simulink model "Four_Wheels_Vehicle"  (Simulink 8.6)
settings: Solver=ode45  StartTime=0.0  StopTime=20  RelTol=1e-3
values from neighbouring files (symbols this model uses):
  beta = 1    [Vehicle_Parameters.m]
  g = 9.81    [Vehicle_Parameters.m]
  H_CoG = 0.700    (= 0.7)    [Vehicle_Parameters.m]
  Hearo = 0.750    (= 0.75)    [Vehicle_Parameters.m]
  Iz = 2480    [Vehicle_Parameters.m]
  Jw = 2.166    [Vehicle_Parameters.m]
  L = 10    [Vehicle_Parameters.m]
  Lf = 1.180    (= 1.18)    [Vehicle_Parameters.m]
  Lr = 1.770    (= 1.77)    [Vehicle_Parameters.m]
  Lw = 1.880    (= 1.88)    [Vehicle_Parameters.m]
  m = 1500    [Vehicle_Parameters.m]
  miu = 0.85    [Vehicle_Parameters.m]
  reff = 0.380    (= 0.38)    [Vehicle_Parameters.m]
undefined symbols (not defined in the file or in its folder): DiscIntNeverNeededParam, Init, Ki, Kp, LowerLimit, sigbuilder_block, Ts, UpperLimit
libraries: simulink x15, powerlib_extras x3
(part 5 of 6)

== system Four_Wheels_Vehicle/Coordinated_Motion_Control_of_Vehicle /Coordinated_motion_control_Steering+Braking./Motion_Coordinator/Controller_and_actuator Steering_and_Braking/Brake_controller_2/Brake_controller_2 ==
  Reference : Inport
  Feedback : Inport  Port=2
  Controller : Subsystem  AncestorBlock=|  DialogController=POWERSYS.PowerSysDialog
      | powerlib_extras/Discrete 
      | Control Blocks/Discrete
      | PI Controller
  Controller1 : Subsystem  AncestorBlock=|  DialogController=POWERSYS.PowerSysDialog
      | powerlib_extras/Discrete 
      | Control Blocks/Discrete
      | PI Controller
  Scope : Scope
  Scope1 : Scope
  Scope2 : Scope  NumInputPorts=2
  Sum1 : Sum  Inputs=-+
  Sum2 : Sum
  Sideslip_Ang : Outport
  Sideslip_Ang1 : Outport  Port=2
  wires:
  Sum2/1 -> Sideslip_Ang1/1, Scope2/2
  Reference/1 -> Sum1/2, Controller1/1(Error)
  Controller1/1(Out) -> Sum2/2
  Feedback/1 -> Sum1/1
  Sum1/1 -> Scope/1, Controller/1(Error)
  Controller/1(Out) -> Sideslip_Ang/1, Scope2/1, Sum2/1, Scope1/1

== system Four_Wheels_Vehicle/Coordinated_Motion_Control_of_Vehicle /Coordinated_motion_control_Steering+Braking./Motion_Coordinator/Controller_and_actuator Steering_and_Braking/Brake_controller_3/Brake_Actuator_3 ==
  input : Inport
  Actuator : Subsystem
  Cut_off_frequency : Constant  Value=10  SampleTime=-1
  output : Outport
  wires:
  input/1 -> Actuator/1(In1)
  Actuator/1(out) -> output/1
  Cut_off_frequency/1 -> Actuator/2(fre)

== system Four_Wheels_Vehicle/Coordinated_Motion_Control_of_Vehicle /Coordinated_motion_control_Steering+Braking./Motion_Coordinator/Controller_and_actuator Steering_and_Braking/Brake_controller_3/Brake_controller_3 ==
  Reference : Inport
  Feedback : Inport  Port=2
  Controller : Subsystem  AncestorBlock=|  DialogController=POWERSYS.PowerSysDialog
      | powerlib_extras/Discrete 
      | Control Blocks/Discrete
      | PI Controller
  Controller1 : Subsystem  AncestorBlock=|  DialogController=POWERSYS.PowerSysDialog
      | powerlib_extras/Discrete 
      | Control Blocks/Discrete
      | PI Controller
  Scope : Scope
  Scope1 : Scope
  Scope2 : Scope  NumInputPorts=2
  Sum1 : Sum  Inputs=-+
  Sum2 : Sum
  Sideslip_Ang : Outport
  Sideslip_Ang1 : Outport  Port=2
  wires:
  Controller/1(Out) -> Scope1/1, Sum2/1, Scope2/1, Sideslip_Ang/1
  Sum1/1 -> Controller/1(Error), Scope/1
  Feedback/1 -> Sum1/1
  Controller1/1(Out) -> Sum2/2
  Reference/1 -> Controller1/1(Error), Sum1/2
  Sum2/1 -> Scope2/2, Sideslip_Ang1/1

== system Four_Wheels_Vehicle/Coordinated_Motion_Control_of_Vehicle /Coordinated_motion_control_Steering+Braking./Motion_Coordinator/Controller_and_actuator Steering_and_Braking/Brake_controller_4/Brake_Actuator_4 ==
  input : Inport
  Actuator : Subsystem
  Cut_off_frequency : Constant  Value=10  SampleTime=-1
  output : Outport
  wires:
  Cut_off_frequency/1 -> Actuator/2(fre)
  Actuator/1(out) -> output/1
  input/1 -> Actuator/1(In1)

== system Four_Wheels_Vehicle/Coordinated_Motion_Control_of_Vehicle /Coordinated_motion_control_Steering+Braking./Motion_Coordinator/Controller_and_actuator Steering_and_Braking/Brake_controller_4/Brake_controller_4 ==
  Reference : Inport
  Feedback : Inport  Port=2
  Controller : Subsystem  AncestorBlock=|  DialogController=POWERSYS.PowerSysDialog
      | powerlib_extras/Discrete 
      | Control Blocks/Discrete
      | PI Controller
  Controller1 : Subsystem  AncestorBlock=|  DialogController=POWERSYS.PowerSysDialog
      | powerlib_extras/Discrete 
      | Control Blocks/Discrete
      | PI Controller
  Scope : Scope
  Scope1 : Scope
  Scope2 : Scope  NumInputPorts=2
  Sum1 : Sum  Inputs=-+
  Sum2 : Sum
  Sideslip_Ang : Outport
  Sideslip_Ang1 : Outport  Port=2
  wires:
  Sum2/1 -> Sideslip_Ang1/1, Scope2/2
  Reference/1 -> Sum1/2, Controller1/1(Error)
  Controller1/1(Out) -> Sum2/2
  Feedback/1 -> Sum1/1
  Sum1/1 -> Scope/1, Controller/1(Error)
  Controller/1(Out) -> Sideslip_Ang/1, Scope2/1, Sum2/1, Scope1/1

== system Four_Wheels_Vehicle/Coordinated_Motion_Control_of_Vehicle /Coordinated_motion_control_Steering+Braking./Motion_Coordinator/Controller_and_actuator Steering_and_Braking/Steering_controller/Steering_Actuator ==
  input : Inport
  Actuator : Subsystem
  Cut_off_frequency : Constant  Value=5  SampleTime=-1
  output : Outport
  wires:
  Cut_off_frequency/1 -> Actuator/2(fre)
  Actuator/1(out) -> output/1
  input/1 -> Actuator/1(In1)

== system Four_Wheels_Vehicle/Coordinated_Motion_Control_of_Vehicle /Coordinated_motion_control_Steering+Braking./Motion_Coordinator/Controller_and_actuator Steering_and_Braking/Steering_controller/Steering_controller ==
  Reference : Inport
  Feedback : Inport  Port=2
  Controller : Subsystem  AncestorBlock=|  DialogController=POWERSYS.PowerSysDialog
      | powerlib_extras/Discrete 
      | Control Blocks/Discrete
      | PI Controller
  Controller1 : Subsystem  AncestorBlock=|  DialogController=POWERSYS.PowerSysDialog
      | powerlib_extras/Discrete 
      | Control Blocks/Discrete
      | PI Controller
  Scope : Scope
  Scope1 : Scope
  Scope2 : Scope  NumInputPorts=2
  Scope3 : Scope  NumInputPorts=2
  Sum1 : Sum  Inputs=-+
  Sum2 : Sum
  Steering_Ang : Outport
  Steering_Ang1 : Outport  Port=2
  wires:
  Feedback/1 -> Sum1/1
  Sum1/1 -> Scope/1, Controller/1(Error)
  Reference/1 -> Scope3/2, Controller1/1(Error), Sum1/2
  Controller/1(Out) -> Sum2/1, Scope2/1, Steering_Ang/1, Scope1/1
  Sum2/1 -> Scope3/1, Scope2/2, Steering_Ang1/1
  Controller1/1(Out) -> Sum2/2

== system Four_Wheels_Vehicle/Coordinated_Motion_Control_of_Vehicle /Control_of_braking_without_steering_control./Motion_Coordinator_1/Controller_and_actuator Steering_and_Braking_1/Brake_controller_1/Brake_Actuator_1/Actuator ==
  In1 : Inport
  fre : Inport  Port=2
  LPF : MATLAB Function  TreatAsAtomicUnit=on
  Unit Delay1 : UnitDelay  SampleTime=1e-3
  out : Outport
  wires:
  fre/1 -> LPF/3(f)
  In1/1 -> LPF/1(in1)
  LPF/1(out) -> Unit Delay1/1, out/1
  Unit Delay1/1 -> LPF/2(in2)

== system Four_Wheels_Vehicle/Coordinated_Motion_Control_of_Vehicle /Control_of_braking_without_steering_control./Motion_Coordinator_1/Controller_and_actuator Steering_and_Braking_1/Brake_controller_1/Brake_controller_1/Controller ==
  note: Discrete PID Controller
  note: Pierre Giroux, Gilbert Sybille Power System Simulation Laboratory IREQ, Hydro-Quebc
  Error : Inport  SampleTime=Ts
  Discrete-Time Integrator : DiscreteIntegrator  InitialCondition=Init  SampleTime=Ts  LimitOutput=on  UpperSaturationLimit=UpperLimit  LowerSaturationLimit=LowerLimit  ICPrevOutput=DiscIntNeverNeededParam  ICPrevScaledInput=DiscIntNeverNeededParam
  Kp4 : Gain  Gain=Kp  SampleTime=Ts
  Kp5 : Gain  Gain=Ki  SampleTime=Ts
  Saturation2 : Saturate  UpperLimit=UpperLimit  LowerLimit=LowerLimit  SampleTime=Ts
  Sum6 : Sum  SampleTime=Ts
  Zero-Order Hold : ZeroOrderHold  SampleTime=Ts
  Out : Outport  SampleTime=Ts  InitialOutput=0
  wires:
  Zero-Order Hold/1 -> Sum6/1
  Saturation2/1 -> Out/1
  Discrete-Time Integrator/1 -> Sum6/2
  Kp4/1 -> Zero-Order Hold/1
  Kp5/1 -> Discrete-Time Integrator/1
  Sum6/1 -> Saturation2/1
  Error/1 -> Kp5/1, Kp4/1

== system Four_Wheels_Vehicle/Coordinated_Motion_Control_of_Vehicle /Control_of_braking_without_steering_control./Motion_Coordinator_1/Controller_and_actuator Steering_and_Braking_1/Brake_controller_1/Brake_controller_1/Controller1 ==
  note: Pierre Giroux, Gilbert Sybille Power System Simulation Laboratory IREQ, Hydro-Quebc
  note: Discrete PID Controller
  Error : Inport  SampleTime=Ts
  Discrete-Time Integrator : DiscreteIntegrator  InitialCondition=Init  SampleTime=Ts  LimitOutput=on  UpperSaturationLimit=UpperLimit  LowerSaturationLimit=LowerLimit  ICPrevOutput=DiscIntNeverNeededParam  ICPrevScaledInput=DiscIntNeverNeededParam
  Kp4 : Gain  Gain=Kp  SampleTime=Ts
  Kp5 : Gain  Gain=Ki  SampleTime=Ts
  Saturation2 : Saturate  UpperLimit=UpperLimit  LowerLimit=LowerLimit  SampleTime=Ts
  Sum6 : Sum  SampleTime=Ts
  Zero-Order Hold : ZeroOrderHold  SampleTime=Ts
  Out : Outport  SampleTime=Ts  InitialOutput=0
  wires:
  Error/1 -> Kp4/1, Kp5/1
  Sum6/1 -> Saturation2/1
  Kp5/1 -> Discrete-Time Integrator/1
  Kp4/1 -> Zero-Order Hold/1
  Discrete-Time Integrator/1 -> Sum6/2
  Saturation2/1 -> Out/1
  Zero-Order Hold/1 -> Sum6/1

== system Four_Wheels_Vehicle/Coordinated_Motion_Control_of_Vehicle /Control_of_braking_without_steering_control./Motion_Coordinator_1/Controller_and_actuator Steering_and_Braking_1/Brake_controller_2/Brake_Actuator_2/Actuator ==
  In1 : Inport
  fre : Inport  Port=2
  LPF : MATLAB Function  TreatAsAtomicUnit=on
  Unit Delay1 : UnitDelay  SampleTime=1e-3
  out : Outport
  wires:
  Unit Delay1/1 -> LPF/2(in2)
  LPF/1(out) -> out/1, Unit Delay1/1
  In1/1 -> LPF/1(in1)
  fre/1 -> LPF/3(f)

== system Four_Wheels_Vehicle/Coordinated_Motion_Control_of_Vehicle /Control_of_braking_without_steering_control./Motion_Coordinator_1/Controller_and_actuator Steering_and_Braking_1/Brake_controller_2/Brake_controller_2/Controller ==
  note: Pierre Giroux, Gilbert Sybille Power System Simulation Laboratory IREQ, Hydro-Quebc
  note: Discrete PID Controller
  Error : Inport  SampleTime=Ts
  Discrete-Time Integrator : DiscreteIntegrator  InitialCondition=Init  SampleTime=Ts  LimitOutput=on  UpperSaturationLimit=UpperLimit  LowerSaturationLimit=LowerLimit  ICPrevOutput=DiscIntNeverNeededParam  ICPrevScaledInput=DiscIntNeverNeededParam
  Kp4 : Gain  Gain=Kp  SampleTime=Ts
  Kp5 : Gain  Gain=Ki  SampleTime=Ts
  Saturation2 : Saturate  UpperLimit=UpperLimit  LowerLimit=LowerLimit  SampleTime=Ts
  Sum6 : Sum  SampleTime=Ts
  Zero-Order Hold : ZeroOrderHold  SampleTime=Ts
  Out : Outport  SampleTime=Ts  InitialOutput=0
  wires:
  Error/1 -> Kp4/1, Kp5/1
  Sum6/1 -> Saturation2/1
  Kp5/1 -> Discrete-Time Integrator/1
  Kp4/1 -> Zero-Order Hold/1
  Discrete-Time Integrator/1 -> Sum6/2
  Saturation2/1 -> Out/1
  Zero-Order Hold/1 -> Sum6/1

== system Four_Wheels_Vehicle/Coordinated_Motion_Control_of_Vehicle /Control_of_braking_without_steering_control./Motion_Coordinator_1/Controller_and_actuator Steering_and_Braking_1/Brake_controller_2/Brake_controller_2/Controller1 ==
  note: Discrete PID Controller
  note: Pierre Giroux, Gilbert Sybille Power System Simulation Laboratory IREQ, Hydro-Quebc
  Error : Inport  SampleTime=Ts
  Discrete-Time Integrator : DiscreteIntegrator  InitialCondition=Init  SampleTime=Ts  LimitOutput=on  UpperSaturationLimit=UpperLimit  LowerSaturationLimit=LowerLimit  ICPrevOutput=DiscIntNeverNeededParam  ICPrevScaledInput=DiscIntNeverNeededParam
  Kp4 : Gain  Gain=Kp  SampleTime=Ts
  Kp5 : Gain  Gain=Ki  SampleTime=Ts
  Saturation2 : Saturate  UpperLimit=UpperLimit  LowerLimit=LowerLimit  SampleTime=Ts
  Sum6 : Sum  SampleTime=Ts
  Zero-Order Hold : ZeroOrderHold  SampleTime=Ts
  Out : Outport  SampleTime=Ts  InitialOutput=0
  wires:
  Zero-Order Hold/1 -> Sum6/1
  Saturation2/1 -> Out/1
  Discrete-Time Integrator/1 -> Sum6/2
  Kp4/1 -> Zero-Order Hold/1
  Kp5/1 -> Discrete-Time Integrator/1
  Sum6/1 -> Saturation2/1
  Error/1 -> Kp5/1, Kp4/1

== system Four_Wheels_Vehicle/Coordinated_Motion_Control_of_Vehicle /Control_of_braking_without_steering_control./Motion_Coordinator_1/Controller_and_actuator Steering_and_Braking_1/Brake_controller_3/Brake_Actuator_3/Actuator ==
  In1 : Inport
  fre : Inport  Port=2
  LPF : MATLAB Function  TreatAsAtomicUnit=on
  Unit Delay1 : UnitDelay  SampleTime=1e-3
  out : Outport
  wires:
  fre/1 -> LPF/3(f)
  In1/1 -> LPF/1(in1)
  LPF/1(out) -> Unit Delay1/1, out/1
  Unit Delay1/1 -> LPF/2(in2)

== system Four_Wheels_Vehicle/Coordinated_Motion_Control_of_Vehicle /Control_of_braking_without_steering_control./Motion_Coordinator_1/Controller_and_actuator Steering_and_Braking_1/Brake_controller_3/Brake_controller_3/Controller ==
  note: Discrete PID Controller
  note: Pierre Giroux, Gilbert Sybille Power System Simulation Laboratory IREQ, Hydro-Quebc
  Error : Inport  SampleTime=Ts
  Discrete-Time Integrator : DiscreteIntegrator  InitialCondition=Init  SampleTime=Ts  LimitOutput=on  UpperSaturationLimit=UpperLimit  LowerSaturationLimit=LowerLimit  ICPrevOutput=DiscIntNeverNeededParam  ICPrevScaledInput=DiscIntNeverNeededParam
  Kp4 : Gain  Gain=Kp  SampleTime=Ts
  Kp5 : Gain  Gain=Ki  SampleTime=Ts
  Saturation2 : Saturate  UpperLimit=UpperLimit  LowerLimit=LowerLimit  SampleTime=Ts
  Sum6 : Sum  SampleTime=Ts
  Zero-Order Hold : ZeroOrderHold  SampleTime=Ts
  Out : Outport  SampleTime=Ts  InitialOutput=0
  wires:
  Zero-Order Hold/1 -> Sum6/1
  Saturation2/1 -> Out/1
  Discrete-Time Integrator/1 -> Sum6/2
  Kp4/1 -> Zero-Order Hold/1
  Kp5/1 -> Discrete-Time Integrator/1
  Sum6/1 -> Saturation2/1
  Error/1 -> Kp5/1, Kp4/1

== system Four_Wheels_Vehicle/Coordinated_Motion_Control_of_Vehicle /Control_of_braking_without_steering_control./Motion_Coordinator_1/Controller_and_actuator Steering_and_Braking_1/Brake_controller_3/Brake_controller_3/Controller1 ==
  note: Pierre Giroux, Gilbert Sybille Power System Simulation Laboratory IREQ, Hydro-Quebc
  note: Discrete PID Controller
  Error : Inport  SampleTime=Ts
  Discrete-Time Integrator : DiscreteIntegrator  InitialCondition=Init  SampleTime=Ts  LimitOutput=on  UpperSaturationLimit=UpperLimit  LowerSaturationLimit=LowerLimit  ICPrevOutput=DiscIntNeverNeededParam  ICPrevScaledInput=DiscIntNeverNeededParam
  Kp4 : Gain  Gain=Kp  SampleTime=Ts
  Kp5 : Gain  Gain=Ki  SampleTime=Ts
  Saturation2 : Saturate  UpperLimit=UpperLimit  LowerLimit=LowerLimit  SampleTime=Ts
  Sum6 : Sum  SampleTime=Ts
  Zero-Order Hold : ZeroOrderHold  SampleTime=Ts
  Out : Outport  SampleTime=Ts  InitialOutput=0
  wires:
  Error/1 -> Kp4/1, Kp5/1
  Sum6/1 -> Saturation2/1
  Kp5/1 -> Discrete-Time Integrator/1
  Kp4/1 -> Zero-Order Hold/1
  Discrete-Time Integrator/1 -> Sum6/2
  Saturation2/1 -> Out/1
  Zero-Order Hold/1 -> Sum6/1

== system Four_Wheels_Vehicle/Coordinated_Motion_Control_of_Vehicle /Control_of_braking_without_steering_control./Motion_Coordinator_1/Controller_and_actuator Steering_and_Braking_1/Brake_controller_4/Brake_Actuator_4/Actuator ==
  In1 : Inport
  fre : Inport  Port=2
  LPF : MATLAB Function  TreatAsAtomicUnit=on
  Unit Delay1 : UnitDelay  SampleTime=1e-3
  out : Outport
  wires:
  Unit Delay1/1 -> LPF/2(in2)
  LPF/1(out) -> out/1, Unit Delay1/1
  In1/1 -> LPF/1(in1)
  fre/1 -> LPF/3(f)

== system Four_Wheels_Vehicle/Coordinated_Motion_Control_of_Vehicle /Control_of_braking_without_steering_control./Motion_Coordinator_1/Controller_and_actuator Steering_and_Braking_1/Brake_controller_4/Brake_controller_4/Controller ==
  note: Pierre Giroux, Gilbert Sybille Power System Simulation Laboratory IREQ, Hydro-Quebc
  note: Discrete PID Controller
  Error : Inport  SampleTime=Ts
  Discrete-Time Integrator : DiscreteIntegrator  InitialCondition=Init  SampleTime=Ts  LimitOutput=on  UpperSaturationLimit=UpperLimit  LowerSaturationLimit=LowerLimit  ICPrevOutput=DiscIntNeverNeededParam  ICPrevScaledInput=DiscIntNeverNeededParam
  Kp4 : Gain  Gain=Kp  SampleTime=Ts
  Kp5 : Gain  Gain=Ki  SampleTime=Ts
  Saturation2 : Saturate  UpperLimit=UpperLimit  LowerLimit=LowerLimit  SampleTime=Ts
  Sum6 : Sum  SampleTime=Ts
  Zero-Order Hold : ZeroOrderHold  SampleTime=Ts
  Out : Outport  SampleTime=Ts  InitialOutput=0
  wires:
  Error/1 -> Kp4/1, Kp5/1
  Sum6/1 -> Saturation2/1
  Kp5/1 -> Discrete-Time Integrator/1
  Kp4/1 -> Zero-Order Hold/1
  Discrete-Time Integrator/1 -> Sum6/2
  Saturation2/1 -> Out/1
  Zero-Order Hold/1 -> Sum6/1

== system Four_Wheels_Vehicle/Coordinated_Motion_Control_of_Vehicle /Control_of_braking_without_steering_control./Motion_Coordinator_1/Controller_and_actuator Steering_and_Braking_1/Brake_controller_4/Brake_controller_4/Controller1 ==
  note: Discrete PID Controller
  note: Pierre Giroux, Gilbert Sybille Power System Simulation Laboratory IREQ, Hydro-Quebc
  Error : Inport  SampleTime=Ts
  Discrete-Time Integrator : DiscreteIntegrator  InitialCondition=Init  SampleTime=Ts  LimitOutput=on  UpperSaturationLimit=UpperLimit  LowerSaturationLimit=LowerLimit  ICPrevOutput=DiscIntNeverNeededParam  ICPrevScaledInput=DiscIntNeverNeededParam
  Kp4 : Gain  Gain=Kp  SampleTime=Ts
  Kp5 : Gain  Gain=Ki  SampleTime=Ts
  Saturation2 : Saturate  UpperLimit=UpperLimit  LowerLimit=LowerLimit  SampleTime=Ts
  Sum6 : Sum  SampleTime=Ts
  Zero-Order Hold : ZeroOrderHold  SampleTime=Ts
  Out : Outport  SampleTime=Ts  InitialOutput=0
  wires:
  Zero-Order Hold/1 -> Sum6/1
  Saturation2/1 -> Out/1
  Discrete-Time Integrator/1 -> Sum6/2
  Kp4/1 -> Zero-Order Hold/1
  Kp5/1 -> Discrete-Time Integrator/1
  Sum6/1 -> Saturation2/1
  Error/1 -> Kp5/1, Kp4/1

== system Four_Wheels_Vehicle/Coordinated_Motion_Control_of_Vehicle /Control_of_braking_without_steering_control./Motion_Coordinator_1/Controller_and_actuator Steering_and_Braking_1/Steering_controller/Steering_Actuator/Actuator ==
  In1 : Inport
  fre : Inport  Port=2
  LPF : MATLAB Function  TreatAsAtomicUnit=on
  Unit Delay1 : UnitDelay  SampleTime=1e-3
  out : Outport
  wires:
  Unit Delay1/1 -> LPF/2(in2)
  LPF/1(out) -> out/1, Unit Delay1/1
  In1/1 -> LPF/1(in1)
  fre/1 -> LPF/3(f)

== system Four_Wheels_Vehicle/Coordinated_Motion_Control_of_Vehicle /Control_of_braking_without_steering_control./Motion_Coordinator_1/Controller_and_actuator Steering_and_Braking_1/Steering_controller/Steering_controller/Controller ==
  note: Pierre Giroux, Gilbert Sybille Power System Simulation Laboratory IREQ, Hydro-Quebc
  note: Discrete PID Controller
  Error : Inport  SampleTime=Ts
  Discrete-Time Integrator : DiscreteIntegrator  InitialCondition=Init  SampleTime=Ts  LimitOutput=on  UpperSaturationLimit=UpperLimit  LowerSaturationLimit=LowerLimit  ICPrevOutput=DiscIntNeverNeededParam  ICPrevScaledInput=DiscIntNeverNeededParam
  Kp4 : Gain  Gain=Kp  SampleTime=Ts
  Kp5 : Gain  Gain=Ki  SampleTime=Ts
  Saturation2 : Saturate  UpperLimit=UpperLimit  LowerLimit=LowerLimit  SampleTime=Ts
  Sum6 : Sum  SampleTime=Ts
  Zero-Order Hold : ZeroOrderHold  SampleTime=Ts
  Out : Outport  SampleTime=Ts  InitialOutput=0
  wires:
  Error/1 -> Kp4/1, Kp5/1
  Sum6/1 -> Saturation2/1
  Kp5/1 -> Discrete-Time Integrator/1
  Kp4/1 -> Zero-Order Hold/1
  Discrete-Time Integrator/1 -> Sum6/2
  Saturation2/1 -> Out/1
  Zero-Order Hold/1 -> Sum6/1

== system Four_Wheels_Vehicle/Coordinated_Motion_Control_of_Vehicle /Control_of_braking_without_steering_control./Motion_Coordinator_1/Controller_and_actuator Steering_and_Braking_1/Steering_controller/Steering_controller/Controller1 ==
  note: Discrete PID Controller
  note: Pierre Giroux, Gilbert Sybille Power System Simulation Laboratory IREQ, Hydro-Quebc
  Error : Inport  SampleTime=Ts
  Discrete-Time Integrator : DiscreteIntegrator  InitialCondition=Init  SampleTime=Ts  LimitOutput=on  UpperSaturationLimit=UpperLimit  LowerSaturationLimit=LowerLimit  ICPrevOutput=DiscIntNeverNeededParam  ICPrevScaledInput=DiscIntNeverNeededParam
  Kp4 : Gain  Gain=Kp  SampleTime=Ts
  Kp5 : Gain  Gain=Ki  SampleTime=Ts
  Saturation2 : Saturate  UpperLimit=UpperLimit  LowerLimit=LowerLimit  SampleTime=Ts
  Sum6 : Sum  SampleTime=Ts
  Zero-Order Hold : ZeroOrderHold  SampleTime=Ts
  Out : Outport  SampleTime=Ts  InitialOutput=0
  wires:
  Zero-Order Hold/1 -> Sum6/1
  Saturation2/1 -> Out/1
  Discrete-Time Integrator/1 -> Sum6/2
  Kp4/1 -> Zero-Order Hold/1
  Kp5/1 -> Discrete-Time Integrator/1
  Sum6/1 -> Saturation2/1
  Error/1 -> Kp5/1, Kp4/1

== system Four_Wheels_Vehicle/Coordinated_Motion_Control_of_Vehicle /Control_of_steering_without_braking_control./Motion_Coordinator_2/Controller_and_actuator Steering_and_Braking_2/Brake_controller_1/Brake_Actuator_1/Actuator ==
  In1 : Inport
  fre : Inport  Port=2
  LPF : MATLAB Function  TreatAsAtomicUnit=on
  Unit Delay1 : UnitDelay  SampleTime=1e-3
  out : Outport
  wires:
  Unit Delay1/1 -> LPF/2(in2)
  LPF/1(out) -> out/1, Unit Delay1/1
  In1/1 -> LPF/1(in1)
  fre/1 -> LPF/3(f)

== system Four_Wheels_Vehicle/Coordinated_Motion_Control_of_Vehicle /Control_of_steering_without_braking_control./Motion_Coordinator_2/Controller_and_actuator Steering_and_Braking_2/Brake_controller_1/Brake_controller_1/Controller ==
  note: Pierre Giroux, Gilbert Sybille Power System Simulation Laboratory IREQ, Hydro-Quebc
  note: Discrete PID Controller
  Error : Inport  SampleTime=Ts
  Discrete-Time Integrator : DiscreteIntegrator  InitialCondition=Init  SampleTime=Ts  LimitOutput=on  UpperSaturationLimit=UpperLimit  LowerSaturationLimit=LowerLimit  ICPrevOutput=DiscIntNeverNeededParam  ICPrevScaledInput=DiscIntNeverNeededParam
  Kp4 : Gain  Gain=Kp  SampleTime=Ts
  Kp5 : Gain  Gain=Ki  SampleTime=Ts
  Saturation2 : Saturate  UpperLimit=UpperLimit  LowerLimit=LowerLimit  SampleTime=Ts
  Sum6 : Sum  SampleTime=Ts
  Zero-Order Hold : ZeroOrderHold  SampleTime=Ts
  Out : Outport  SampleTime=Ts  InitialOutput=0
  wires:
  Error/1 -> Kp4/1, Kp5/1
  Sum6/1 -> Saturation2/1
  Kp5/1 -> Discrete-Time Integrator/1
  Kp4/1 -> Zero-Order Hold/1
  Discrete-Time Integrator/1 -> Sum6/2
  Saturation2/1 -> Out/1
  Zero-Order Hold/1 -> Sum6/1

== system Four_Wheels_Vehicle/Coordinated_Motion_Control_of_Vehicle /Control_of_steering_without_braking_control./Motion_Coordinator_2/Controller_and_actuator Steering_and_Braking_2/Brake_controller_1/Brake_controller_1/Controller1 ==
  note: Discrete PID Controller
  note: Pierre Giroux, Gilbert Sybille Power System Simulation Laboratory IREQ, Hydro-Quebc
  Error : Inport  SampleTime=Ts
  Discrete-Time Integrator : DiscreteIntegrator  InitialCondition=Init  SampleTime=Ts  LimitOutput=on  UpperSaturationLimit=UpperLimit  LowerSaturationLimit=LowerLimit  ICPrevOutput=DiscIntNeverNeededParam  ICPrevScaledInput=DiscIntNeverNeededParam
  Kp4 : Gain  Gain=Kp  SampleTime=Ts
  Kp5 : Gain  Gain=Ki  SampleTime=Ts
  Saturation2 : Saturate  UpperLimit=UpperLimit  LowerLimit=LowerLimit  SampleTime=Ts
  Sum6 : Sum  SampleTime=Ts
  Zero-Order Hold : ZeroOrderHold  SampleTime=Ts
  Out : Outport  SampleTime=Ts  InitialOutput=0
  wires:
  Zero-Order Hold/1 -> Sum6/1
  Saturation2/1 -> Out/1
  Discrete-Time Integrator/1 -> Sum6/2
  Kp4/1 -> Zero-Order Hold/1
  Kp5/1 -> Discrete-Time Integrator/1
  Sum6/1 -> Saturation2/1
  Error/1 -> Kp5/1, Kp4/1

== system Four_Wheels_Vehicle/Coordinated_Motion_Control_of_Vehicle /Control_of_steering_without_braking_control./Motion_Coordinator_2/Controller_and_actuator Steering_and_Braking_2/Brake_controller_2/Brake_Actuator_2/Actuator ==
  In1 : Inport
  fre : Inport  Port=2
  LPF : MATLAB Function  TreatAsAtomicUnit=on
  Unit Delay1 : UnitDelay  SampleTime=1e-3
  out : Outport
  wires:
  fre/1 -> LPF/3(f)
  In1/1 -> LPF/1(in1)
  LPF/1(out) -> Unit Delay1/1, out/1
  Unit Delay1/1 -> LPF/2(in2)

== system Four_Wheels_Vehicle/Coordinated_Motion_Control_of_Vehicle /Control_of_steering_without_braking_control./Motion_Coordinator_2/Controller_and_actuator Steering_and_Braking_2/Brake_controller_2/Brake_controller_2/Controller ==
  note: Discrete PID Controller
  note: Pierre Giroux, Gilbert Sybille Power System Simulation Laboratory IREQ, Hydro-Quebc
  Error : Inport  SampleTime=Ts
  Discrete-Time Integrator : DiscreteIntegrator  InitialCondition=Init  SampleTime=Ts  LimitOutput=on  UpperSaturationLimit=UpperLimit  LowerSaturationLimit=LowerLimit  ICPrevOutput=DiscIntNeverNeededParam  ICPrevScaledInput=DiscIntNeverNeededParam
  Kp4 : Gain  Gain=Kp  SampleTime=Ts
  Kp5 : Gain  Gain=Ki  SampleTime=Ts
  Saturation2 : Saturate  UpperLimit=UpperLimit  LowerLimit=LowerLimit  SampleTime=Ts
  Sum6 : Sum  SampleTime=Ts
  Zero-Order Hold : ZeroOrderHold  SampleTime=Ts
  Out : Outport  SampleTime=Ts  InitialOutput=0
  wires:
  Zero-Order Hold/1 -> Sum6/1
  Saturation2/1 -> Out/1
  Discrete-Time Integrator/1 -> Sum6/2
  Kp4/1 -> Zero-Order Hold/1
  Kp5/1 -> Discrete-Time Integrator/1
  Sum6/1 -> Saturation2/1
  Error/1 -> Kp5/1, Kp4/1

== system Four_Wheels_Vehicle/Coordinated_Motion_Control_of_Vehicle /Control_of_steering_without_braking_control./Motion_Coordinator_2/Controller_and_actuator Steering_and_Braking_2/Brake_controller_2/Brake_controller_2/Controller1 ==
  note: Pierre Giroux, Gilbert Sybille Power System Simulation Laboratory IREQ, Hydro-Quebc
  note: Discrete PID Controller
  Error : Inport  SampleTime=Ts
  Discrete-Time Integrator : DiscreteIntegrator  InitialCondition=Init  SampleTime=Ts  LimitOutput=on  UpperSaturationLimit=UpperLimit  LowerSaturationLimit=LowerLimit  ICPrevOutput=DiscIntNeverNeededParam  ICPrevScaledInput=DiscIntNeverNeededParam
  Kp4 : Gain  Gain=Kp  SampleTime=Ts
  Kp5 : Gain  Gain=Ki  SampleTime=Ts
  Saturation2 : Saturate  UpperLimit=UpperLimit  LowerLimit=LowerLimit  SampleTime=Ts
  Sum6 : Sum  SampleTime=Ts
  Zero-Order Hold : ZeroOrderHold  SampleTime=Ts
  Out : Outport  SampleTime=Ts  InitialOutput=0
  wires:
  Error/1 -> Kp4/1, Kp5/1
  Sum6/1 -> Saturation2/1
  Kp5/1 -> Discrete-Time Integrator/1
  Kp4/1 -> Zero-Order Hold/1
  Discrete-Time Integrator/1 -> Sum6/2
  Saturation2/1 -> Out/1
  Zero-Order Hold/1 -> Sum6/1

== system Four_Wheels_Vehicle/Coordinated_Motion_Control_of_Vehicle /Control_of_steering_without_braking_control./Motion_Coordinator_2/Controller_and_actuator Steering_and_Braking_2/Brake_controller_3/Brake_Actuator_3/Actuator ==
  In1 : Inport
  fre : Inport  Port=2
  LPF : MATLAB Function  TreatAsAtomicUnit=on
  Unit Delay1 : UnitDelay  SampleTime=1e-3
  out : Outport
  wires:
  Unit Delay1/1 -> LPF/2(in2)
  LPF/1(out) -> out/1, Unit Delay1/1
  In1/1 -> LPF/1(in1)
  fre/1 -> LPF/3(f)

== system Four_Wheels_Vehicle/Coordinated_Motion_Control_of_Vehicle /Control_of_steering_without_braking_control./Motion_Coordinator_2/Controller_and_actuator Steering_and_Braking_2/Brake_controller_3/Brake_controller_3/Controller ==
  note: Pierre Giroux, Gilbert Sybille Power System Simulation Laboratory IREQ, Hydro-Quebc
  note: Discrete PID Controller
  Error : Inport  SampleTime=Ts
  Discrete-Time Integrator : DiscreteIntegrator  InitialCondition=Init  SampleTime=Ts  LimitOutput=on  UpperSaturationLimit=UpperLimit  LowerSaturationLimit=LowerLimit  ICPrevOutput=DiscIntNeverNeededParam  ICPrevScaledInput=DiscIntNeverNeededParam
  Kp4 : Gain  Gain=Kp  SampleTime=Ts
  Kp5 : Gain  Gain=Ki  SampleTime=Ts
  Saturation2 : Saturate  UpperLimit=UpperLimit  LowerLimit=LowerLimit  SampleTime=Ts
  Sum6 : Sum  SampleTime=Ts
  Zero-Order Hold : ZeroOrderHold  SampleTime=Ts
  Out : Outport  SampleTime=Ts  InitialOutput=0
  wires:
  Error/1 -> Kp4/1, Kp5/1
  Sum6/1 -> Saturation2/1
  Kp5/1 -> Discrete-Time Integrator/1
  Kp4/1 -> Zero-Order Hold/1
  Discrete-Time Integrator/1 -> Sum6/2
  Saturation2/1 -> Out/1
  Zero-Order Hold/1 -> Sum6/1

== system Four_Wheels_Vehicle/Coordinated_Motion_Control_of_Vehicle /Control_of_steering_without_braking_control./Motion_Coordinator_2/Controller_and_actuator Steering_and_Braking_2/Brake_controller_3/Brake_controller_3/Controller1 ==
  note: Discrete PID Controller
  note: Pierre Giroux, Gilbert Sybille Power System Simulation Laboratory IREQ, Hydro-Quebc
  Error : Inport  SampleTime=Ts
  Discrete-Time Integrator : DiscreteIntegrator  InitialCondition=Init  SampleTime=Ts  LimitOutput=on  UpperSaturationLimit=UpperLimit  LowerSaturationLimit=LowerLimit  ICPrevOutput=DiscIntNeverNeededParam  ICPrevScaledInput=DiscIntNeverNeededParam
  Kp4 : Gain  Gain=Kp  SampleTime=Ts
  Kp5 : Gain  Gain=Ki  SampleTime=Ts
  Saturation2 : Saturate  UpperLimit=UpperLimit  LowerLimit=LowerLimit  SampleTime=Ts
  Sum6 : Sum  SampleTime=Ts
  Zero-Order Hold : ZeroOrderHold  SampleTime=Ts
  Out : Outport  SampleTime=Ts  InitialOutput=0
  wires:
  Zero-Order Hold/1 -> Sum6/1
  Saturation2/1 -> Out/1
  Discrete-Time Integrator/1 -> Sum6/2
  Kp4/1 -> Zero-Order Hold/1
  Kp5/1 -> Discrete-Time Integrator/1
  Sum6/1 -> Saturation2/1
  Error/1 -> Kp5/1, Kp4/1

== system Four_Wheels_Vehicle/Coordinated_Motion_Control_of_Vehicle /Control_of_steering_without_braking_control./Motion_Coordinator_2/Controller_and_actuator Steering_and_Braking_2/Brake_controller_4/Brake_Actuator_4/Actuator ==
  In1 : Inport
  fre : Inport  Port=2
  LPF : MATLAB Function  TreatAsAtomicUnit=on
  Unit Delay1 : UnitDelay  SampleTime=1e-3
  out : Outport
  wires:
  fre/1 -> LPF/3(f)
  In1/1 -> LPF/1(in1)
  LPF/1(out) -> Unit Delay1/1, out/1
  Unit Delay1/1 -> LPF/2(in2)

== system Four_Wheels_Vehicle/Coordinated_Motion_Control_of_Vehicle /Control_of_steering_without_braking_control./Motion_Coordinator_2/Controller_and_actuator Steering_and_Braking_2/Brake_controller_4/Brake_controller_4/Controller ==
  note: Discrete PID Controller
  note: Pierre Giroux, Gilbert Sybille Power System Simulation Laboratory IREQ, Hydro-Quebc
  Error : Inport  SampleTime=Ts
  Discrete-Time Integrator : DiscreteIntegrator  InitialCondition=Init  SampleTime=Ts  LimitOutput=on  UpperSaturationLimit=UpperLimit  LowerSaturationLimit=LowerLimit  ICPrevOutput=DiscIntNeverNeededParam  ICPrevScaledInput=DiscIntNeverNeededParam
  Kp4 : Gain  Gain=Kp  SampleTime=Ts
  Kp5 : Gain  Gain=Ki  SampleTime=Ts
  Saturation2 : Saturate  UpperLimit=UpperLimit  LowerLimit=LowerLimit  SampleTime=Ts
  Sum6 : Sum  SampleTime=Ts
  Zero-Order Hold : ZeroOrderHold  SampleTime=Ts
  Out : Outport  SampleTime=Ts  InitialOutput=0
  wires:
  Zero-Order Hold/1 -> Sum6/1
  Saturation2/1 -> Out/1
  Discrete-Time Integrator/1 -> Sum6/2
  Kp4/1 -> Zero-Order Hold/1
  Kp5/1 -> Discrete-Time Integrator/1
  Sum6/1 -> Saturation2/1
  Error/1 -> Kp5/1, Kp4/1

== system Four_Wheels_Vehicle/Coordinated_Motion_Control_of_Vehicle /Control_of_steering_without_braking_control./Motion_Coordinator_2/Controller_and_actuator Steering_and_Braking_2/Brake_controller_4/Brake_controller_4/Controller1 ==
  note: Pierre Giroux, Gilbert Sybille Power System Simulation Laboratory IREQ, Hydro-Quebc
  note: Discrete PID Controller
  Error : Inport  SampleTime=Ts
  Discrete-Time Integrator : DiscreteIntegrator  InitialCondition=Init  SampleTime=Ts  LimitOutput=on  UpperSaturationLimit=UpperLimit  LowerSaturationLimit=LowerLimit  ICPrevOutput=DiscIntNeverNeededParam  ICPrevScaledInput=DiscIntNeverNeededParam
  Kp4 : Gain  Gain=Kp  SampleTime=Ts
  Kp5 : Gain  Gain=Ki  SampleTime=Ts
  Saturation2 : Saturate  UpperLimit=UpperLimit  LowerLimit=LowerLimit  SampleTime=Ts
  Sum6 : Sum  SampleTime=Ts
  Zero-Order Hold : ZeroOrderHold  SampleTime=Ts
  Out : Outport  SampleTime=Ts  InitialOutput=0
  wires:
  Error/1 -> Kp4/1, Kp5/1
  Sum6/1 -> Saturation2/1
  Kp5/1 -> Discrete-Time Integrator/1
  Kp4/1 -> Zero-Order Hold/1
  Discrete-Time Integrator/1 -> Sum6/2
  Saturation2/1 -> Out/1
  Zero-Order Hold/1 -> Sum6/1

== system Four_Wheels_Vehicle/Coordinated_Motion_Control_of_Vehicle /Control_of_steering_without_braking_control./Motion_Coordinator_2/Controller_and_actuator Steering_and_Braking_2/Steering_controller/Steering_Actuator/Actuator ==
  In1 : Inport
  fre : Inport  Port=2
  LPF : MATLAB Function  TreatAsAtomicUnit=on
  Unit Delay1 : UnitDelay  SampleTime=1e-3
  out : Outport
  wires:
  fre/1 -> LPF/3(f)
  In1/1 -> LPF/1(in1)
  LPF/1(out) -> Unit Delay1/1, out/1
  Unit Delay1/1 -> LPF/2(in2)

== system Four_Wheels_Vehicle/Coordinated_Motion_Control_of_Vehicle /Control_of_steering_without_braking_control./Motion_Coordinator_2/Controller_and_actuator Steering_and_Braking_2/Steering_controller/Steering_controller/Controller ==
  note: Discrete PID Controller
  note: Pierre Giroux, Gilbert Sybille Power System Simulation Laboratory IREQ, Hydro-Quebc
  Error : Inport  SampleTime=Ts
  Discrete-Time Integrator : DiscreteIntegrator  InitialCondition=Init  SampleTime=Ts  LimitOutput=on  UpperSaturationLimit=UpperLimit  LowerSaturationLimit=LowerLimit  ICPrevOutput=DiscIntNeverNeededParam  ICPrevScaledInput=DiscIntNeverNeededParam
  Kp4 : Gain  Gain=Kp  SampleTime=Ts
  Kp5 : Gain  Gain=Ki  SampleTime=Ts
  Saturation2 : Saturate  UpperLimit=UpperLimit  LowerLimit=LowerLimit  SampleTime=Ts
  Sum6 : Sum  SampleTime=Ts
  Zero-Order Hold : ZeroOrderHold  SampleTime=Ts
  Out : Outport  SampleTime=Ts  InitialOutput=0
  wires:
  Zero-Order Hold/1 -> Sum6/1
  Saturation2/1 -> Out/1
  Discrete-Time Integrator/1 -> Sum6/2
  Kp4/1 -> Zero-Order Hold/1
  Kp5/1 -> Discrete-Time Integrator/1
  Sum6/1 -> Saturation2/1
  Error/1 -> Kp5/1, Kp4/1

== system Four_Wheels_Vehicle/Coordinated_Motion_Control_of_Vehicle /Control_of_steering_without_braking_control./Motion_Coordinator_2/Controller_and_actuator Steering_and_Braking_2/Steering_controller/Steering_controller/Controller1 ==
  note: Pierre Giroux, Gilbert Sybille Power System Simulation Laboratory IREQ, Hydro-Quebc
  note: Discrete PID Controller
  Error : Inport  SampleTime=Ts
  Discrete-Time Integrator : DiscreteIntegrator  InitialCondition=Init  SampleTime=Ts  LimitOutput=on  UpperSaturationLimit=UpperLimit  LowerSaturationLimit=LowerLimit  ICPrevOutput=DiscIntNeverNeededParam  ICPrevScaledInput=DiscIntNeverNeededParam
  Kp4 : Gain  Gain=Kp  SampleTime=Ts
  Kp5 : Gain  Gain=Ki  SampleTime=Ts
  Saturation2 : Saturate  UpperLimit=UpperLimit  LowerLimit=LowerLimit  SampleTime=Ts
  Sum6 : Sum  SampleTime=Ts
  Zero-Order Hold : ZeroOrderHold  SampleTime=Ts
  Out : Outport  SampleTime=Ts  InitialOutput=0
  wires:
  Error/1 -> Kp4/1, Kp5/1
  Sum6/1 -> Saturation2/1
  Kp5/1 -> Discrete-Time Integrator/1
  Kp4/1 -> Zero-Order Hold/1
  Discrete-Time Integrator/1 -> Sum6/2
  Saturation2/1 -> Out/1
  Zero-Order Hold/1 -> Sum6/1

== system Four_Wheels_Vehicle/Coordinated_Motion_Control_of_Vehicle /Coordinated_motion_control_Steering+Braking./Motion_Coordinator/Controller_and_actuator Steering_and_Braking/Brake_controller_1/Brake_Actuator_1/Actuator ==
  In1 : Inport
  fre : Inport  Port=2
  LPF : MATLAB Function  TreatAsAtomicUnit=on
  Unit Delay1 : UnitDelay  SampleTime=1e-3
  out : Outport
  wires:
  Unit Delay1/1 -> LPF/2(in2)
  LPF/1(out) -> out/1, Unit Delay1/1
  In1/1 -> LPF/1(in1)
  fre/1 -> LPF/3(f)

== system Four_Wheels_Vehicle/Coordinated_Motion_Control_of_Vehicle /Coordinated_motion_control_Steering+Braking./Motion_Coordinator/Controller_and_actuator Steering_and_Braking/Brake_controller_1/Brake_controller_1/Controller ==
  note: Pierre Giroux, Gilbert Sybille Power System Simulation Laboratory IREQ, Hydro-Quebc
  note: Discrete PID Controller
  Error : Inport  SampleTime=Ts
  Discrete-Time Integrator : DiscreteIntegrator  InitialCondition=Init  SampleTime=Ts  LimitOutput=on  UpperSaturationLimit=UpperLimit  LowerSaturationLimit=LowerLimit  ICPrevOutput=DiscIntNeverNeededParam  ICPrevScaledInput=DiscIntNeverNeededParam
  Kp4 : Gain  Gain=Kp  SampleTime=Ts
  Kp5 : Gain  Gain=Ki  SampleTime=Ts
  Saturation2 : Saturate  UpperLimit=UpperLimit  LowerLimit=LowerLimit  SampleTime=Ts
  Sum6 : Sum  SampleTime=Ts
  Zero-Order Hold : ZeroOrderHold  SampleTime=Ts
  Out : Outport  SampleTime=Ts  InitialOutput=0
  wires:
  Error/1 -> Kp4/1, Kp5/1
  Sum6/1 -> Saturation2/1
  Kp5/1 -> Discrete-Time Integrator/1
  Kp4/1 -> Zero-Order Hold/1
  Discrete-Time Integrator/1 -> Sum6/2
  Saturation2/1 -> Out/1
  Zero-Order Hold/1 -> Sum6/1

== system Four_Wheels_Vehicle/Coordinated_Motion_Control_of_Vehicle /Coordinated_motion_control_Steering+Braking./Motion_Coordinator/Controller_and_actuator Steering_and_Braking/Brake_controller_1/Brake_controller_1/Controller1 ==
  note: Discrete PID Controller
  note: Pierre Giroux, Gilbert Sybille Power System Simulation Laboratory IREQ, Hydro-Quebc
  Error : Inport  SampleTime=Ts
  Discrete-Time Integrator : DiscreteIntegrator  InitialCondition=Init  SampleTime=Ts  LimitOutput=on  UpperSaturationLimit=UpperLimit  LowerSaturationLimit=LowerLimit  ICPrevOutput=DiscIntNeverNeededParam  ICPrevScaledInput=DiscIntNeverNeededParam
  Kp4 : Gain  Gain=Kp  SampleTime=Ts
  Kp5 : Gain  Gain=Ki  SampleTime=Ts
  Saturation2 : Saturate  UpperLimit=UpperLimit  LowerLimit=LowerLimit  SampleTime=Ts
  Sum6 : Sum  SampleTime=Ts
  Zero-Order Hold : ZeroOrderHold  SampleTime=Ts
  Out : Outport  SampleTime=Ts  InitialOutput=0
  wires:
  Zero-Order Hold/1 -> Sum6/1
  Saturation2/1 -> Out/1
  Discrete-Time Integrator/1 -> Sum6/2
  Kp4/1 -> Zero-Order Hold/1
  Kp5/1 -> Discrete-Time Integrator/1
  Sum6/1 -> Saturation2/1
  Error/1 -> Kp5/1, Kp4/1

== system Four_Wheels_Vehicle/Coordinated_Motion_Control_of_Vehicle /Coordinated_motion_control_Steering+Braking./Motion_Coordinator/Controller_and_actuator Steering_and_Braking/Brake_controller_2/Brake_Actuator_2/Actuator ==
  In1 : Inport
  fre : Inport  Port=2
  LPF : MATLAB Function  TreatAsAtomicUnit=on
  Unit Delay1 : UnitDelay  SampleTime=1e-3
  out : Outport
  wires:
  fre/1 -> LPF/3(f)
  In1/1 -> LPF/1(in1)
  LPF/1(out) -> Unit Delay1/1, out/1
  Unit Delay1/1 -> LPF/2(in2)

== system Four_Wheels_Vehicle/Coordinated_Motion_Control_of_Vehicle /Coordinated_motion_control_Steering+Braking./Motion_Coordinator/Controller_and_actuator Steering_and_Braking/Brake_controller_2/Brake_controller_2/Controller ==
  note: Discrete PID Controller
  note: Pierre Giroux, Gilbert Sybille Power System Simulation Laboratory IREQ, Hydro-Quebc
  Error : Inport  SampleTime=Ts
  Discrete-Time Integrator : DiscreteIntegrator  InitialCondition=Init  SampleTime=Ts  LimitOutput=on  UpperSaturationLimit=UpperLimit  LowerSaturationLimit=LowerLimit  ICPrevOutput=DiscIntNeverNeededParam  ICPrevScaledInput=DiscIntNeverNeededParam
  Kp4 : Gain  Gain=Kp  SampleTime=Ts
  Kp5 : Gain  Gain=Ki  SampleTime=Ts
  Saturation2 : Saturate  UpperLimit=UpperLimit  LowerLimit=LowerLimit  SampleTime=Ts
  Sum6 : Sum  SampleTime=Ts
  Zero-Order Hold : ZeroOrderHold  SampleTime=Ts
  Out : Outport  SampleTime=Ts  InitialOutput=0
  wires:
  Zero-Order Hold/1 -> Sum6/1
  Saturation2/1 -> Out/1
  Discrete-Time Integrator/1 -> Sum6/2
  Kp4/1 -> Zero-Order Hold/1
  Kp5/1 -> Discrete-Time Integrator/1
  Sum6/1 -> Saturation2/1
  Error/1 -> Kp5/1, Kp4/1

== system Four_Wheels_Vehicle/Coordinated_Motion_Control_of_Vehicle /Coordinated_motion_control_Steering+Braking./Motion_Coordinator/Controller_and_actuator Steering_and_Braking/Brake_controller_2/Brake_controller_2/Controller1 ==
  note: Pierre Giroux, Gilbert Sybille Power System Simulation Laboratory IREQ, Hydro-Quebc
  note: Discrete PID Controller
  Error : Inport  SampleTime=Ts
  Discrete-Time Integrator : DiscreteIntegrator  InitialCondition=Init  SampleTime=Ts  LimitOutput=on  UpperSaturationLimit=UpperLimit  LowerSaturationLimit=LowerLimit  ICPrevOutput=DiscIntNeverNeededParam  ICPrevScaledInput=DiscIntNeverNeededParam
  Kp4 : Gain  Gain=Kp  SampleTime=Ts
  Kp5 : Gain  Gain=Ki  SampleTime=Ts
  Saturation2 : Saturate  UpperLimit=UpperLimit  LowerLimit=LowerLimit  SampleTime=Ts
  Sum6 : Sum  SampleTime=Ts
  Zero-Order Hold : ZeroOrderHold  SampleTime=Ts
  Out : Outport  SampleTime=Ts  InitialOutput=0
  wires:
  Error/1 -> Kp4/1, Kp5/1
  Sum6/1 -> Saturation2/1
  Kp5/1 -> Discrete-Time Integrator/1
  Kp4/1 -> Zero-Order Hold/1
  Discrete-Time Integrator/1 -> Sum6/2
  Saturation2/1 -> Out/1
  Zero-Order Hold/1 -> Sum6/1

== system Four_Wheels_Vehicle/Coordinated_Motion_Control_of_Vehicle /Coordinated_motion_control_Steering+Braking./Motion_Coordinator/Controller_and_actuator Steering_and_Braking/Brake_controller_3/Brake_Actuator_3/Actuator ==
  In1 : Inport
  fre : Inport  Port=2
  LPF : MATLAB Function  TreatAsAtomicUnit=on
  Unit Delay1 : UnitDelay  SampleTime=1e-3
  out : Outport
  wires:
  Unit Delay1/1 -> LPF/2(in2)
  LPF/1(out) -> out/1, Unit Delay1/1
  In1/1 -> LPF/1(in1)
  fre/1 -> LPF/3(f)

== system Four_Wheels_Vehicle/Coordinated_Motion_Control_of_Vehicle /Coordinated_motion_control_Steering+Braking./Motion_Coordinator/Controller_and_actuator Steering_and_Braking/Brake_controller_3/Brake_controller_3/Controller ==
  note: Pierre Giroux, Gilbert Sybille Power System Simulation Laboratory IREQ, Hydro-Quebc
  note: Discrete PID Controller
  Error : Inport  SampleTime=Ts
  Discrete-Time Integrator : DiscreteIntegrator  InitialCondition=Init  SampleTime=Ts  LimitOutput=on  UpperSaturationLimit=UpperLimit  LowerSaturationLimit=LowerLimit  ICPrevOutput=DiscIntNeverNeededParam  ICPrevScaledInput=DiscIntNeverNeededParam
  Kp4 : Gain  Gain=Kp  SampleTime=Ts
  Kp5 : Gain  Gain=Ki  SampleTime=Ts
  Saturation2 : Saturate  UpperLimit=UpperLimit  LowerLimit=LowerLimit  SampleTime=Ts
  Sum6 : Sum  SampleTime=Ts
  Zero-Order Hold : ZeroOrderHold  SampleTime=Ts
  Out : Outport  SampleTime=Ts  InitialOutput=0
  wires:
  Error/1 -> Kp4/1, Kp5/1
  Sum6/1 -> Saturation2/1
  Kp5/1 -> Discrete-Time Integrator/1
  Kp4/1 -> Zero-Order Hold/1
  Discrete-Time Integrator/1 -> Sum6/2
  Saturation2/1 -> Out/1
  Zero-Order Hold/1 -> Sum6/1

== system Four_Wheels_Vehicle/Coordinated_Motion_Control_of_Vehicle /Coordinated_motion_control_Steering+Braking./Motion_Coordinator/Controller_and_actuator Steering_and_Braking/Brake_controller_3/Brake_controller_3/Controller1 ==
  note: Discrete PID Controller
  note: Pierre Giroux, Gilbert Sybille Power System Simulation Laboratory IREQ, Hydro-Quebc
  Error : Inport  SampleTime=Ts
  Discrete-Time Integrator : DiscreteIntegrator  InitialCondition=Init  SampleTime=Ts  LimitOutput=on  UpperSaturationLimit=UpperLimit  LowerSaturationLimit=LowerLimit  ICPrevOutput=DiscIntNeverNeededParam  ICPrevScaledInput=DiscIntNeverNeededParam
  Kp4 : Gain  Gain=Kp  SampleTime=Ts
  Kp5 : Gain  Gain=Ki  SampleTime=Ts
  Saturation2 : Saturate  UpperLimit=UpperLimit  LowerLimit=LowerLimit  SampleTime=Ts
  Sum6 : Sum  SampleTime=Ts
  Zero-Order Hold : ZeroOrderHold  SampleTime=Ts
  Out : Outport  SampleTime=Ts  InitialOutput=0
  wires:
  Zero-Order Hold/1 -> Sum6/1
  Saturation2/1 -> Out/1
  Discrete-Time Integrator/1 -> Sum6/2
  Kp4/1 -> Zero-Order Hold/1
  Kp5/1 -> Discrete-Time Integrator/1
  Sum6/1 -> Saturation2/1
  Error/1 -> Kp5/1, Kp4/1

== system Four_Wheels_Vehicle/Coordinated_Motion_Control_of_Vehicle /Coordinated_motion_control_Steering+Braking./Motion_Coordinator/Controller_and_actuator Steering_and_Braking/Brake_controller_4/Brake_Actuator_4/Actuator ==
  In1 : Inport
  fre : Inport  Port=2
  LPF : MATLAB Function  TreatAsAtomicUnit=on
  Unit Delay1 : UnitDelay  SampleTime=1e-3
  out : Outport
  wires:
  fre/1 -> LPF/3(f)
  In1/1 -> LPF/1(in1)
  LPF/1(out) -> Unit Delay1/1, out/1
  Unit Delay1/1 -> LPF/2(in2)

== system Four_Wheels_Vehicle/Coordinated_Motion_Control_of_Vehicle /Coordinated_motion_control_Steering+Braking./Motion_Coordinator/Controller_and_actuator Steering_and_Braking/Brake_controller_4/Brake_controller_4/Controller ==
  note: Discrete PID Controller
  note: Pierre Giroux, Gilbert Sybille Power System Simulation Laboratory IREQ, Hydro-Quebc
  Error : Inport  SampleTime=Ts
  Discrete-Time Integrator : DiscreteIntegrator  InitialCondition=Init  SampleTime=Ts  LimitOutput=on  UpperSaturationLimit=UpperLimit  LowerSaturationLimit=LowerLimit  ICPrevOutput=DiscIntNeverNeededParam  ICPrevScaledInput=DiscIntNeverNeededParam
  Kp4 : Gain  Gain=Kp  SampleTime=Ts
  Kp5 : Gain  Gain=Ki  SampleTime=Ts
  Saturation2 : Saturate  UpperLimit=UpperLimit  LowerLimit=LowerLimit  SampleTime=Ts
  Sum6 : Sum  SampleTime=Ts
  Zero-Order Hold : ZeroOrderHold  SampleTime=Ts
  Out : Outport  SampleTime=Ts  InitialOutput=0
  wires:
  Zero-Order Hold/1 -> Sum6/1
  Saturation2/1 -> Out/1
  Discrete-Time Integrator/1 -> Sum6/2
  Kp4/1 -> Zero-Order Hold/1
  Kp5/1 -> Discrete-Time Integrator/1
  Sum6/1 -> Saturation2/1
  Error/1 -> Kp5/1, Kp4/1

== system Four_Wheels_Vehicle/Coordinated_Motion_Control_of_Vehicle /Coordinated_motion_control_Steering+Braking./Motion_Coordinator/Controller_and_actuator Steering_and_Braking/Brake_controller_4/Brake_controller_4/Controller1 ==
  note: Pierre Giroux, Gilbert Sybille Power System Simulation Laboratory IREQ, Hydro-Quebc
  note: Discrete PID Controller
  Error : Inport  SampleTime=Ts
  Discrete-Time Integrator : DiscreteIntegrator  InitialCondition=Init  SampleTime=Ts  LimitOutput=on  UpperSaturationLimit=UpperLimit  LowerSaturationLimit=LowerLimit  ICPrevOutput=DiscIntNeverNeededParam  ICPrevScaledInput=DiscIntNeverNeededParam
  Kp4 : Gain  Gain=Kp  SampleTime=Ts
  Kp5 : Gain  Gain=Ki  SampleTime=Ts
  Saturation2 : Saturate  UpperLimit=UpperLimit  LowerLimit=LowerLimit  SampleTime=Ts
  Sum6 : Sum  SampleTime=Ts
  Zero-Order Hold : ZeroOrderHold  SampleTime=Ts
  Out : Outport  SampleTime=Ts  InitialOutput=0
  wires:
  Error/1 -> Kp4/1, Kp5/1
  Sum6/1 -> Saturation2/1
  Kp5/1 -> Discrete-Time Integrator/1
  Kp4/1 -> Zero-Order Hold/1
  Discrete-Time Integrator/1 -> Sum6/2
  Saturation2/1 -> Out/1
  Zero-Order Hold/1 -> Sum6/1

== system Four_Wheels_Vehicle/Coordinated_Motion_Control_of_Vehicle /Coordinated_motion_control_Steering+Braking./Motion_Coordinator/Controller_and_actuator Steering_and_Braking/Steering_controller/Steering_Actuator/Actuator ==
  In1 : Inport
  fre : Inport  Port=2
  LPF : MATLAB Function  TreatAsAtomicUnit=on
  Unit Delay1 : UnitDelay  SampleTime=1e-3
  out : Outport
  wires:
  fre/1 -> LPF/3(f)
  In1/1 -> LPF/1(in1)
  LPF/1(out) -> Unit Delay1/1, out/1
  Unit Delay1/1 -> LPF/2(in2)

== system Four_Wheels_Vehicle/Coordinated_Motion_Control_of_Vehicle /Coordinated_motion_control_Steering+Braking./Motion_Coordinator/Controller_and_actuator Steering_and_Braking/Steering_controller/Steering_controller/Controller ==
  note: Discrete PID Controller
  note: Pierre Giroux, Gilbert Sybille Power System Simulation Laboratory IREQ, Hydro-Quebc
  Error : Inport  SampleTime=Ts
  Discrete-Time Integrator : DiscreteIntegrator  InitialCondition=Init  SampleTime=Ts  LimitOutput=on  UpperSaturationLimit=UpperLimit  LowerSaturationLimit=LowerLimit  ICPrevOutput=DiscIntNeverNeededParam  ICPrevScaledInput=DiscIntNeverNeededParam
  Kp4 : Gain  Gain=Kp  SampleTime=Ts
  Kp5 : Gain  Gain=Ki  SampleTime=Ts
  Saturation2 : Saturate  UpperLimit=UpperLimit  LowerLimit=LowerLimit  SampleTime=Ts
  Sum6 : Sum  SampleTime=Ts
  Zero-Order Hold : ZeroOrderHold  SampleTime=Ts
  Out : Outport  SampleTime=Ts  InitialOutput=0
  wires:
  Zero-Order Hold/1 -> Sum6/1
  Saturation2/1 -> Out/1
  Discrete-Time Integrator/1 -> Sum6/2
  Kp4/1 -> Zero-Order Hold/1
  Kp5/1 -> Discrete-Time Integrator/1
  Sum6/1 -> Saturation2/1
  Error/1 -> Kp5/1, Kp4/1

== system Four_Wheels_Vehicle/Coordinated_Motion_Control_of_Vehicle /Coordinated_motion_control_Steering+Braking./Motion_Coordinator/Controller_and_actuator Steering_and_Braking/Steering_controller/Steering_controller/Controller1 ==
  note: Pierre Giroux, Gilbert Sybille Power System Simulation Laboratory IREQ, Hydro-Quebc
  note: Discrete PID Controller
  Error : Inport  SampleTime=Ts
  Discrete-Time Integrator : DiscreteIntegrator  InitialCondition=Init  SampleTime=Ts  LimitOutput=on  UpperSaturationLimit=UpperLimit  LowerSaturationLimit=LowerLimit  ICPrevOutput=DiscIntNeverNeededParam  ICPrevScaledInput=DiscIntNeverNeededParam
  Kp4 : Gain  Gain=Kp  SampleTime=Ts
  Kp5 : Gain  Gain=Ki  SampleTime=Ts
  Saturation2 : Saturate  UpperLimit=UpperLimit  LowerLimit=LowerLimit  SampleTime=Ts
  Sum6 : Sum  SampleTime=Ts
  Zero-Order Hold : ZeroOrderHold  SampleTime=Ts
  Out : Outport  SampleTime=Ts  InitialOutput=0
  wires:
  Error/1 -> Kp4/1, Kp5/1
  Sum6/1 -> Saturation2/1
  Kp5/1 -> Discrete-Time Integrator/1
  Kp4/1 -> Zero-Order Hold/1
  Discrete-Time Integrator/1 -> Sum6/2
  Saturation2/1 -> Out/1
  Zero-Order Hold/1 -> Sum6/1

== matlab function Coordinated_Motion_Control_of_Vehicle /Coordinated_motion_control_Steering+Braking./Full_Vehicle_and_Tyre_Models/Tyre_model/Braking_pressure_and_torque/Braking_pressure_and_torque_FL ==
% ================================================================================
% Function: Dugoff_Tire_FL
% Version:  0.00
% Since:    24 May 2016
% Author:   T.C. Lin
% Input:	Sigma, Fz_FL, alpha_FL, miu
% Output:	Fx_FL, Fy_FL
% Timing:   TBD
% Description: NA
% ================================================================================

function [P_FL, Tb_FL]  = Dugoff_Tire_FL(M, reff, tw, SteeringAng)
%# codegen

% Brake gain
Kb = 100;

% Dugoff's tire model with a variable lamda in the wheel model
P_FL = -2*M*reff/(Kb*tw)*cos(SteeringAng);

Tb_FL=Kb*P_FL;

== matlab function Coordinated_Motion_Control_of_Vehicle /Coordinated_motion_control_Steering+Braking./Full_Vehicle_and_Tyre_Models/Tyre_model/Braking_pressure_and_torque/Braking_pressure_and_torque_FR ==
% ================================================================================
% Function: Dugoff_Tire_FL
% Version:  0.00
% Since:    24 May 2016
% Author:   T.C. Lin
% Input:	Sigma, Fz_FL, alpha_FL, miu
% Output:	Fx_FL, Fy_FL
% Timing:   TBD
% Description: NA
% ================================================================================

function [P_FR, Tb_FR] = Dugoff_Tire_FL(M, reff, tw, SteeringAng)
%# codegen

% Brake gain
Kb = 100;

% Dugoff's tire model with a variable lamda in the wheel model
P_FR = 2*M*reff/(Kb*tw)*cos(SteeringAng);

Tb_FR=Kb*P_FR;
